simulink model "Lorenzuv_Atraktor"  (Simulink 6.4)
settings: Solver=ode45  StartTime=0.0  StopTime=200  MaxStep=0.005  RelTol=1e-5

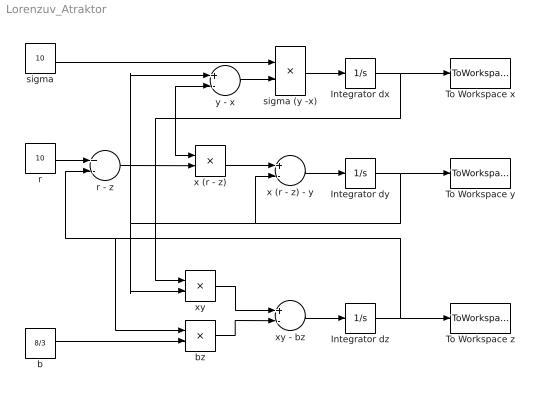
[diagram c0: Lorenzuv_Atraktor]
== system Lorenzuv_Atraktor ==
  Integrator dx : Integrator  InitialCondition=20
  Integrator dy : Integrator  InitialCondition=5
  Integrator dz : Integrator  InitialCondition=-5
  To Workspace x : ToWorkspace  VariableName=x  SampleTime=-1  SaveFormat=Structure With Time
  To Workspace y : ToWorkspace  VariableName=y  SampleTime=-1  SaveFormat=Structure With Time
  To Workspace z : ToWorkspace  VariableName=z  SampleTime=-1  SaveFormat=Structure With Time
  b : Constant  Value=8/3  OutDataType=sfix(16)  ConRadixGroup=Use specified scaling  OutScaling=2^0  SampleTime=inf  FramePeriod=inf
  bz : Product
  r : Constant  Value=10  OutDataType=sfix(16)  ConRadixGroup=Use specified scaling  OutScaling=2^0  SampleTime=inf  FramePeriod=inf
  r - z : Sum  Inputs=+-  OutScaling=2^-10
  sigma : Constant  Value=10  OutDataType=sfix(16)  ConRadixGroup=Use specified scaling  OutScaling=2^0  SampleTime=inf  FramePeriod=inf
  sigma (y -x) : Product
  x (r - z) : Product
  x (r - z) - y : Sum  Inputs=+-  OutScaling=2^-10
  xy : Product
  xy - bz : Sum  Inputs=+-  OutScaling=2^-10
  y - x : Sum  Inputs=+-  OutScaling=2^-10
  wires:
  Integrator dz/1 -> To Workspace z/1, bz/1, r - z/2
  Integrator dy/1 -> x (r - z) - y/2, y - x/1, xy/2, To Workspace y/1
  Integrator dx/1 -> x (r - z)/1, y - x/2, xy/1, To Workspace x/1
  x (r - z) - y/1 -> Integrator dy/1
  x (r - z)/1 -> x (r - z) - y/1
  r - z/1 -> x (r - z)/2
  r/1 -> r - z/1
  sigma (y -x)/1 -> Integrator dx/1
  y - x/1 -> sigma (y -x)/2
  sigma/1 -> sigma (y -x)/1
  xy - bz/1 -> Integrator dz/1
  bz/1 -> xy - bz/2
  xy/1 -> xy - bz/1
  b/1 -> bz/2
